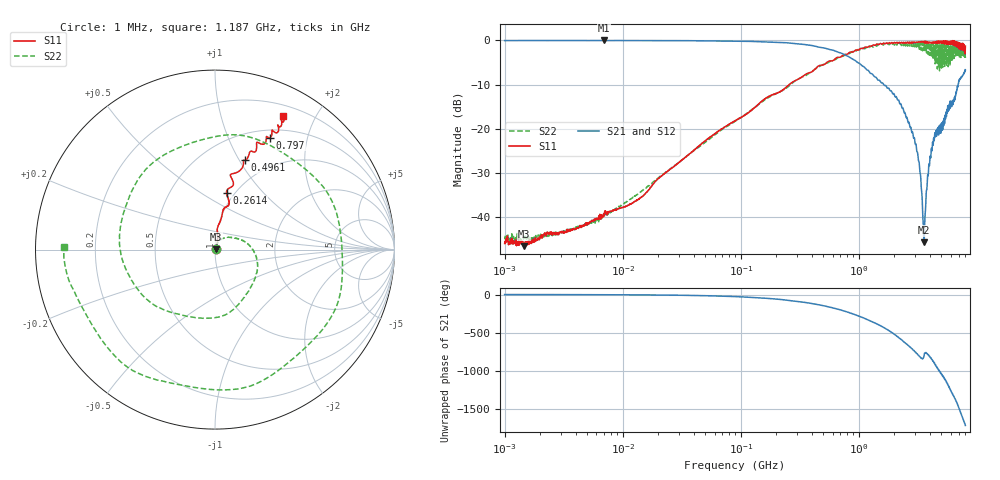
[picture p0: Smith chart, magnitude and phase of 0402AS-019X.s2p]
!s-Parameter Generated by FASTRON Sdn. Bhd.
!FASTRON P/N : 0402AS-019X
!Keysight Technologies: E5071C_MY46733604_B.14.02
!Date: Mon Dec 01 10:32:07 2025
!Version  :Rev00  Mon Dec 01 10:32:07 2025
!Data & Calibration Information:
!Freq  S11:SOLT2(ON)  S21:SOLT2(ON)  S12:SOLT2(ON)  S22:SOLT2(ON)
!PortZ  Port1:50+j0  Port2:50+j0
!When reading reference impedance value at option line is always used.
! Remarks : This data is being provided solely for informational purposes.
# Hz S dB R 50
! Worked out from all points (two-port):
!   1601 points, 1 MHz to 8 GHz, reference 50 ohm
!   highest |S21| = -0.04 dB at 6.912 MHz (marker M1); lowest = -45.6 dB at 3.568 GHz (marker M2)
!   |S21| within 3 dB of the highest: start of sweep to 730 MHz
!   lowest |S11| = -46.5 dB at 1.468 MHz (marker M3), VSWR 1.01, Z = 50.4 + j0.256 ohm
!   |S11| at or under -10 dB: start of sweep to 256.8 MHz
!   |S22| runs from -45.8 to -0.3 dB; largest |S21 - S12| = 0.016
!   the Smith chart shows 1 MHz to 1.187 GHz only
!   S11 on the Smith chart (normalised r, x): 1 MHz: 1.01, +0.01; 261.4 MHz: 0.92, +0.65; 496.1 MHz: 0.77, +1.06; 797 MHz: 0.59, +1.44; 1.187 GHz: 0.32, +1.58
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1000000  -45.90 31.9  -0.06 -0.3  -0.04 -0.4  -44.30 22.8
1468277  -46.50 32.4  -0.06 -0.5  -0.04 -0.5  -44.40 12.9
4479405  -41.90 49.7  -0.06 -1.4  -0.04 -1.4  -41.90 49.9
6911657  -39.20 46.7  -0.04 -2.2  -0.05 -2.2  -39.10 50.9
2.00676e7  -31.20 69.5  -0.07 -6.2  -0.06 -6.1  -31.10 69.8
8.994653e7  -18.10 83.5  -0.18 -27.2  -0.16 -27.2  -18.30 32.5
2.614059e8  -9.86 78.4  -0.63 -77.7  -0.62 -77.7  -10.10 -58.5
4.006501e8  -7.10 75.1  -1.18 -118.0  -1.17 -118.0  -6.97 -134.0
4.96067e8  -5.58 71.4  -1.69 -145.0  -1.68 -144.0  -5.50 178.0
7.969768e8  -3.15 63.8  -3.54 132.0  -3.52 132.0  -3.02 20.3
1.002268e9  -2.12 61.9  -5.15 78.5  -5.14 78.5  -2.12 -86.4
1.187136e9  -1.57 63.1  -6.73 32.5  -6.72 32.5  -1.49 179.0
1.542898e9  -0.77 70.4  -9.53 -51.4  -9.53 -51.4  -0.97 3.1
1.7949e9  -0.60 75.8  -10.80 -110.0  -10.90 -110.0  -0.94 -119.0
2.082516e9  -0.55 81.9  -12.80 -179.0  -12.80 -179.0  -0.93 99.0
2.457552e9  -0.65 87.1  -16.30 92.9  -16.30 93.0  -0.66 -83.7
2.824359e9  -0.60 96.0  -20.90 12.3  -20.80 12.3  -0.52 99.9
3.203473e9  -0.38 105.0  -27.20 -72.1  -27.10 -72.2  -0.70 -88.2
3.568312e9  -0.22 118.0  -45.60 -78.4  -45.60 -78.6  -2.29 75.0
3.95342e9  -0.41 122.0  -28.30 -86.8  -28.30 -87.1  -3.35 -102.0
4.296652e9  -0.52 130.0  -22.20 -155.0  -22.30 -155.0  -0.48 108.0
8e9  -1.32 -107.0  -6.69 90.6  -6.74 91.0  -3.95 125.0
